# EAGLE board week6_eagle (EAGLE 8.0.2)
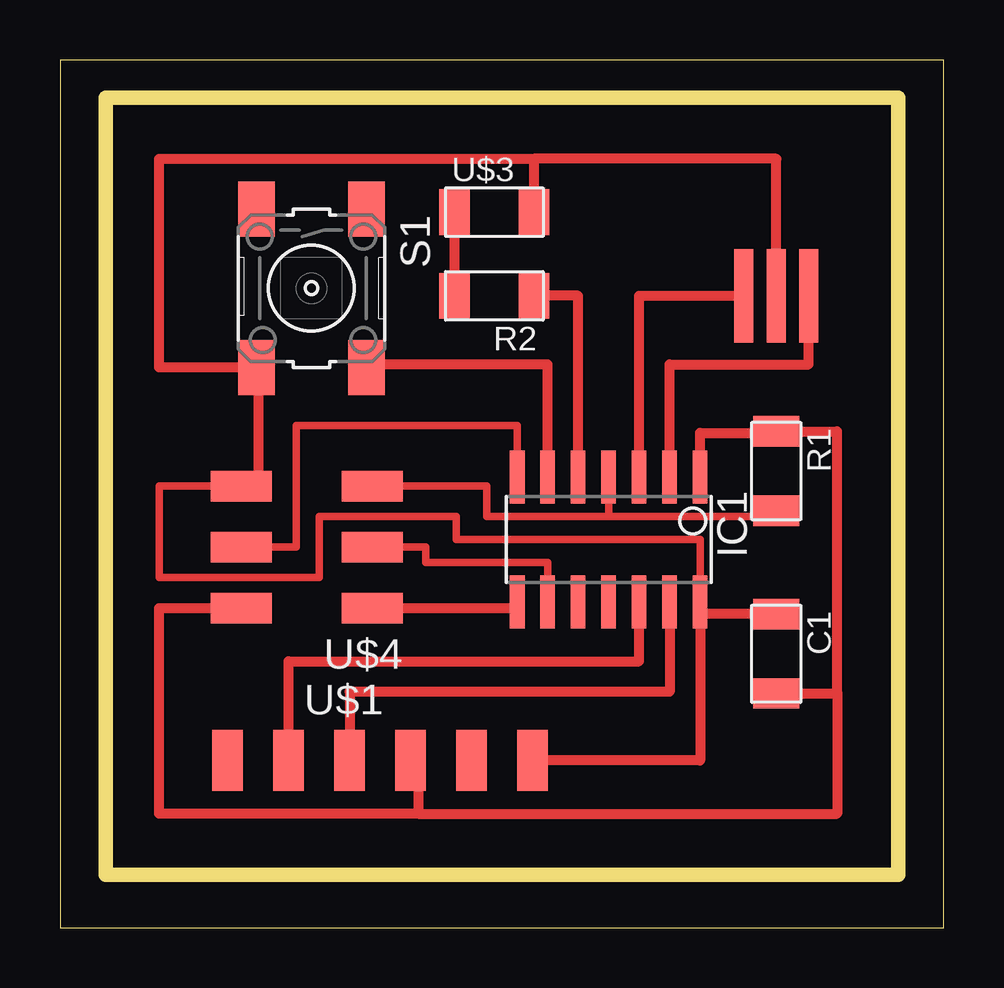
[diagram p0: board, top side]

Size 36.82 x 36.19 mm. Coordinates in mm from the lower left corner, seen from the top.
Outline: 0,0 36.82,0 36.82,36.19 0,36.19 0,0
Outline: 1.91,34.61 34.92,34.61 34.92,2.22 1.91,2.22 1.91,34.61
Copper layers (1*16): Top 0.035mm / dielectric 1.5mm / Bottom 0.035mm
Design rules "default": minimum track width 10mil, minimum drill 24mil, track to track 8mil, track to pad 8mil, pad to pad 8mil, via to via 8mil, smd to smd 8mil, copper to edge 40mil, drill to drill 8mil, minimum pad ring 10mil, minimum via ring 8mil, stop-mask expansion 4mil, vias tented up to drill 0mil, thermal gap 10mil

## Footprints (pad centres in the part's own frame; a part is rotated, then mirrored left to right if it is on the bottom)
C1206FAB = smd 1.27 x 1.905: 1 -1.651,0; 2 1.651,0
SOIC14 = smd 0.61 x 2.21: 1 -3.81,-2.603; 2 -2.54,-2.603; 3 -1.27,-2.603; 4 0,-2.603; 5 1.27,-2.603; 6 2.54,-2.603; 7 3.81,-2.603; 8 3.81,2.603; 9 2.54,2.603; 10 1.27,2.603; 11 0,2.603; 12 -1.27,2.603; 13 -2.54,2.603; 14 -3.81,2.603
R1206FAB = smd 1.27 x 1.905: 1 -1.651,0; 2 1.651,0
6MM_SWITCH = smd 2.286 x 1.524: 1 -3.302,2.286; 2 3.302,2.286; 3 -3.302,-2.286; 4 3.302,-2.286
1X06SMD = smd 2.54 x 1.27: 1 0,6.35; 2 0,3.81; 3 0,1.27; 4 0,-1.27; 5 0,-3.81; 6 0,-6.35
EFOBM = smd 0.8 x 3.9: 1 -1.35,0; 2 0,0; 3 1.35,0
LED1206FAB = smd 1.27 x 1.905: 1 -1.651,0; 2 1.651,0
2X03SMD = smd 2.54 x 1.27: 1 -2.54,2.54; 2 2.92,2.54; 3 -2.54,0; 4 2.92,0; 5 -2.54,-2.54; 6 2.92,-2.54

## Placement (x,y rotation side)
C1  [C1206FAB]  29.84,11.43 270 top
IC1  ATTINY44-SSU  [SOIC14]  22.86,16.19 180 top
R1  [R1206FAB]  29.84,19.05 270 top
R2  330  [R1206FAB]  18.1,26.35 180 top
S1  [6MM_SWITCH]  10.48,26.67 270 top
U$1  FTDI-SMD-HEADER  [1X06SMD]  13.34,6.99 270 top
U$2  RESONATOR  [EFOBM]  29.84,26.35 0 top
U$3  LEDFAB1206  [LED1206FAB]  18.1,29.84 0 top
U$4  AVRISPSMD  [2X03SMD]  10.48,15.88 180 top

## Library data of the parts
C1 IC1 R1 R2 S1 U$1-U$4 = fab

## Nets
BOTON: IC1.6 S1.2
GND: C1.1 IC1.14 S1.4 U$1.1 U$2.2 U$3.2 U$4.6
LED: IC1.5 R2.1
MISO: IC1.8 U$4.1
MOSI: IC1.7 U$4.4
N$1: R2.2 U$3.1
N$2: IC1.3 U$2.1
N$3: IC1.2 U$2.3
RST: IC1.4 R1.2 U$4.5
RXD: IC1.12 U$1.5
SCK: IC1.9 U$4.3
TXD: IC1.13 U$1.4
VCC: C1.2 IC1.1 R1.1 U$1.3 U$4.2

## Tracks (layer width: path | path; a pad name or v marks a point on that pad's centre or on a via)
BOTON
  Top 0.406: IC1.6 20.32,23.5 12.76,23.5 S1.2
GND
  Top 0.305: U$4.6 4.13,18.41 4.13,14.61 10.79,14.61 10.79,17.15 16.51,17.15 16.51,16.19 26.67,16.19 IC1.14
  Top 0.406: 8.26,18.73 8.26,18.41 U$4.6 7.56,18.73 8.26,18.73 | 8.26,18.73 8.26,23.37 S1.4 4.13,23.37 4.13,32.07 19.75,32.07 | 19.75,32.07 U$3.2 | U$2.2 29.84,32.07 19.75,32.07 | IC1.14 26.67,13.08 | 26.67,13.08 26.67,6.99 U$1.1 | C1.1 26.67,13.08
LED
  Top 0.406: R2.1 21.59,26.35 IC1.5
MISO
  Top 0.406: 19.05,13.33 IC1.8 19.05,13.33 | U$4.1 19.05,13.33
MOSI
  Top 0.305: U$4.4 9.84,15.88 9.84,20.96 19.05,20.96 IC1.7
N$1
  Top 0.406: R2.2 U$3.1
N$2
  Top 0.406: IC1.3 24.13,26.35 U$2.1
N$3
  Top 0.406: IC1.2 25.4,23.5 31.2,23.5 U$2.3
RST
  Top 0.305: U$4.5 17.78,18.41 17.78,17.15 22.86,17.15 | 22.86,17.15 29.84,17.15 R1.2 | IC1.4 22.86,17.15
RXD
  Top 0.406: IC1.12 24.13,11.11 9.53,11.11 U$1.5
SCK
  Top 0.305: IC1.9 20.32,15.24 15.24,15.24 15.24,15.88 U$4.3
TXD
  Top 0.406: IC1.13 25.4,9.84 12.07,9.84 U$1.4
VCC
  Top 0.406: 7.62,13.33 U$4.2 4.13,13.33 4.13,4.76 14.92,4.76 | 32.39,9.84 32.39,20.7 R1.1 29.84,20.64 26.67,20.64 IC1.1 | 32.39,9.84 32.39,4.76 14.92,4.76 | U$1.3 14.92,6.99 14.92,4.76 | C1.2 32.39,9.78 32.39,9.84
